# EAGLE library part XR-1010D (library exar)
Second order switched capacitor FILTER
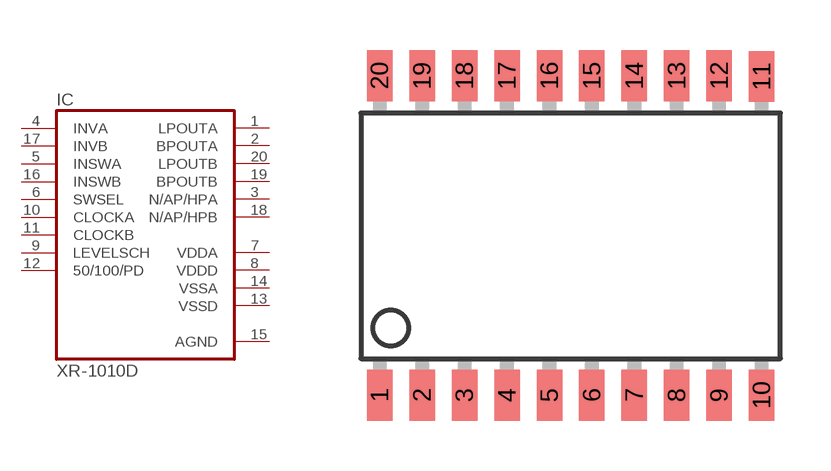
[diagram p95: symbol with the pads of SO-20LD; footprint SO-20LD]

Designator prefix IC

## XR-1010D (OC_FARNELL: unknown; OC_NEWARK: unknown)  [SO-20LD]
1  LPOUTA  out
2  BPOUTA  out
3  N/AP/HPA  out
4  INVA  in
5  INSWA  in
6  SWSEL  in
7  VDDA  pwr
8  VDDD  pwr
9  LEVELSCH  in
10  CLOCKA  in
11  CLOCKB  in
12  50/100/PD  in
13  VSSD  pwr
14  VSSA  pwr
15  AGND  pwr
16  INSWB  in
17  INVB  in
18  N/AP/HPB  out
19  BPOUTB  out
20  LPOUTB  out

## Footprint SO-20LD (pad centres in mm)
Small Outline Package
smd 0.762 x 1.524: 1 -5.715,-4.775; 2 -4.445,-4.775; 3 -3.175,-4.775; 4 -1.905,-4.775; 5 -0.635,-4.775; 6 0.635,-4.775; 7 1.905,-4.775; 8 3.175,-4.775; 9 4.445,-4.775; 10 5.715,-4.775; 11 5.715,4.75; 12 4.445,4.775; 13 3.175,4.775; 14 1.905,4.775; 15 0.635,4.775; 16 -0.635,4.775; 17 -1.905,4.775; 18 -3.175,4.775; 19 -4.445,4.775; 20 -5.715,4.775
